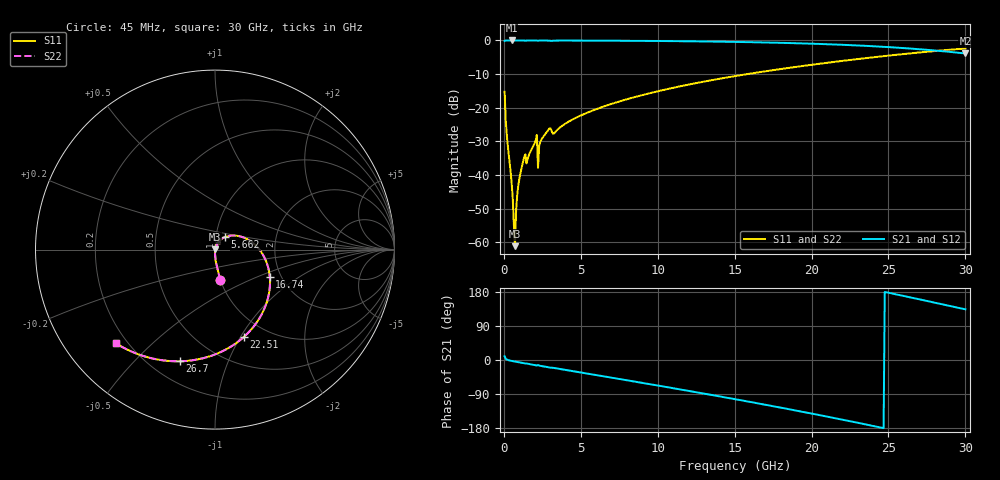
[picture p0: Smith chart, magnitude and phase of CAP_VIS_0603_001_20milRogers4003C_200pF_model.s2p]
! S-parameter model data by Modelithics Inc.  support@modelithics.com  813-866-6335  Tampa FL USA
! S-Parameter data specifications:
! Substrate: 20-mil Rogers 4003C, substrate thickness, H=0.508mm, Dielectric constant, Er=3.75
! PCB Mounting Pad Footprint: Pad width, PadW=0.90mm , Pad length, PadL=1.00mm , Pad gap, PadG (edge-to-edge)=1.00mm , Reference planes=3.0mm apart
! Created Wed Nov 18 13:32:58 2015
# hz S ma R 50
! 2 Port Network Data from SP1.SP block
! freq  magS11  angS11  magS21  angS21  magS12  angS12  magS22  angS22
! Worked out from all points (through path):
!   401 points, 45 MHz to 30 GHz, reference 50 ohm
!   highest |S21| = 0.00 dB at 494.3 MHz (marker M1); lowest = -3.9 dB at 30 GHz (marker M2)
!   group delay of S21, straight-line fit = 20.9 ps
!   lowest |S11| = -61.1 dB at 719 MHz (marker M3), VSWR 1.00, Z = 50.1 + j0.0654 ohm
!   |S11| at or under -10 dB: start of sweep to 15.81 GHz
!   |S22| runs from -61.1 to -2.4 dB; largest |S21 - S12| = 0
!   S11 on the Smith chart (normalised r, x): 45 MHz: 1.00, -0.35; 5.662 GHz: 1.11, +0.16; 16.74 GHz: 1.75, -0.60; 22.51 GHz: 0.78, -1.03; 26.7 GHz: 0.32, -0.68; 30 GHz: 0.16, -0.39
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4.5e7  0.1731 -80.2  0.9847 9.7  0.9847 9.7  0.1731 -80.2
4.94325e8  0.008067 -89.1  0.9995 -2.4  0.9995 -2.4  0.008067 -89.1
5.692125e8  0.004734 -87.1  0.9995 -3.0  0.9995 -3.0  0.004734 -87.1
7.189875e8  0.0008817 47.8  0.9994 -4.2  0.9994 -4.2  0.0008817 47.8
7.93875e8  0.003061 74.5  0.9994 -4.7  0.9994 -4.7  0.003061 74.5
1.018538e9  0.009235 79.4  0.9992 -6.4  0.9992 -6.4  0.009235 79.4
1.2432e9  0.01562 77.7  0.9986 -8.0  0.9986 -8.0  0.01562 77.7
1.992075e9  0.02959 74.6  0.9982 -13.1  0.9982 -13.1  0.02959 74.6
2.366512e9  0.03126 72.3  0.998 -15.4  0.998 -15.4  0.03126 72.3
2.4414e9  0.03385 71.8  0.9979 -16.0  0.9979 -16.0  0.03385 71.8
2.890725e9  0.04717 65.1  0.994 -19.3  0.994 -19.3  0.04717 65.1
3.34005e9  0.04363 62.5  0.9944 -21.6  0.9944 -21.6  0.04363 62.5
5.062462e9  0.078 55.4  0.995 -33.5  0.995 -33.5  0.078 55.4
5.661562e9  0.08903 51.5  0.994 -37.5  0.994 -37.5  0.08903 51.5
1.007992e10  0.1775 21.5  0.9812 -67.9  0.9812 -67.9  0.1775 21.5
1.50225e10  0.2956 -13.8  0.9514 -103.3  0.9514 -103.3  0.2956 -13.8
1.674491e10  0.3415 -26.6  0.9356 -116.2  0.9356 -116.2  0.3415 -26.6
2.003996e10  0.4364 -52.0  0.8946 -141.6  0.8946 -141.6  0.4364 -52.0
2.251125e10  0.5134 -72.0  0.8522 -161.6  0.8522 -161.6  0.5134 -72.0
2.505742e10  0.5973 -93.3  0.7952 177.0  0.7952 177.0  0.5973 -93.3
2.670495e10  0.6527 -107.6  0.75 162.8  0.75 162.8  0.6527 -107.6
3e10  0.7603 -136.7  0.6403 133.7  0.6403 133.7  0.7603 -136.7
